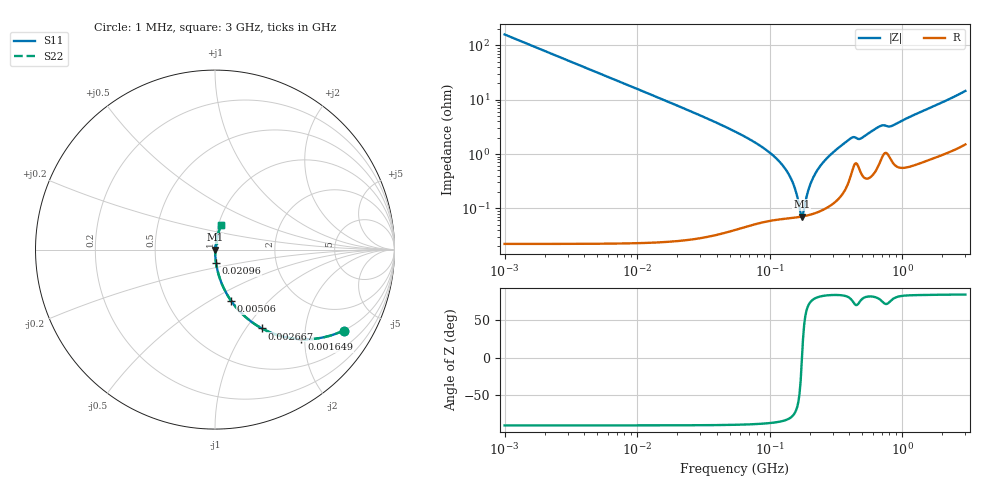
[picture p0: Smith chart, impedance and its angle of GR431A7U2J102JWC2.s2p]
!Murata Part Number: GR431A7U2J102JWC2
!These Parameters are Measured in Series Mode Connection
!Data Generated on Jun 10, 2025
!  o--ll--o
!Port1  Port2
!  o------o
!Operation Temp=25[degC], DC Bias Voltage=0[V]
!Freq. Start=1000[kHz] Stop=3[GHz] 401[Steps]
# Hz S RI R 50
!Freq.(Hz) S11(Real) S11(Imag) S21(Real) S21(Imag) S12(Real) S12(Imag) S22(Real) S22(Imag)
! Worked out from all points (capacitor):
!   401 points, 1 MHz to 3 GHz, reference 50 ohm
!   read as one part in series: C = 1 nF near 1.041 MHz
!   lowest |Z| = 70.9 mohm at 174.9 MHz (marker M1)
!   series resonance near 175.4 MHz, so ESL is about 820 pH
!   S11 on the Smith chart (normalised r, x): 1 MHz: 1.00, -3.18; 1.649 MHz: 1.00, -1.93; 2.667 MHz: 1.00, -1.19; 5.06 MHz: 1.00, -0.63; 20.96 MHz: 1.00, -0.15; 3 GHz: 1.03, +0.29
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1000000  0.7162 -0.4507  0.2838 0.4507  0.2838 0.4507  0.7162 -0.4507
1649378  0.4813 -0.4995  0.5187 0.4995  0.5187 0.4995  0.4813 -0.4995
2666535  0.262 -0.4395  0.738 0.4395  0.738 0.4395  0.262 -0.4395
3823119  0.1473 -0.3541  0.8527 0.3541  0.8527 0.3541  0.1473 -0.3541
5059610  0.0898 -0.2855  0.9102 0.2855  0.9102 0.2855  0.0898 -0.2855
1.461624e7  0.0117 -0.1066  0.9883 0.1066  0.9883 0.1066  0.0117 -0.1066
2.095589e7  0.00579 -0.0742  0.9942 0.0742  0.9942 0.0742  0.00579 -0.0742
5.477226e7  0.00107 -0.026  0.9989 0.026  0.9989 0.026  0.00107 -0.026
9.034013e7  0.000722 -0.0128  0.9993 0.0128  0.9993 0.0128  0.000722 -0.0128
1.244416e8  0.000675 -0.0063  0.9993 0.0063  0.9993 0.0063  0.000675 -0.0063
1.49005e8  0.000677 -0.00296  0.9993 0.00296  0.9993 0.00296  0.000677 -0.00296
1.680187e8  0.000696 -0.000777  0.9993 0.000777  0.9993 0.000777  0.000696 -0.000777
1.748812e8  0.000707 -4.95e-05  0.9993 4.95e-05  0.9993 4.95e-05  0.000707 -4.95e-05
1.820241e8  0.000721 0.00068  0.9993 -0.00068  0.9993 -0.00068  0.000721 0.00068
1.971969e8  0.000758 0.00215  0.9992 -0.00215  0.9992 -0.00215  0.000758 0.00215
2.094008e8  0.000795 0.00327  0.9992 -0.00327  0.9992 -0.00327  0.000795 0.00327
2.609752e8  0.00103 0.00757  0.999 -0.00757  0.999 -0.00757  0.00103 0.00757
3.973271e8  0.00352 0.0181  0.9965 -0.0181  0.9965 -0.0181  0.00352 0.0181
4.853736e8  0.00498 0.0185  0.995 -0.0185  0.995 -0.0185  0.00498 0.0185
6.958997e8  0.00902 0.0318  0.991 -0.0318  0.991 -0.0318  0.00902 0.0318
8.005644e8  0.0097 0.0303  0.9903 -0.0303  0.9903 -0.0303  0.0097 0.0303
3e9  0.0344 0.1375  0.9656 -0.1375  0.9656 -0.1375  0.0344 0.1375
